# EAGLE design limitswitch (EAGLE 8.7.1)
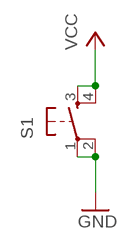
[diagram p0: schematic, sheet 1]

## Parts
S1  6MM_SWITCH6MM_SWITCH  [6MM_SWITCH]

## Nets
GND: S1.1(P) S1.2(P1)
VCC: S1.3(S) S1.4(S1)

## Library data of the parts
S1 = fab.lbr:6MM_SWITCH: OMRON SWITCH

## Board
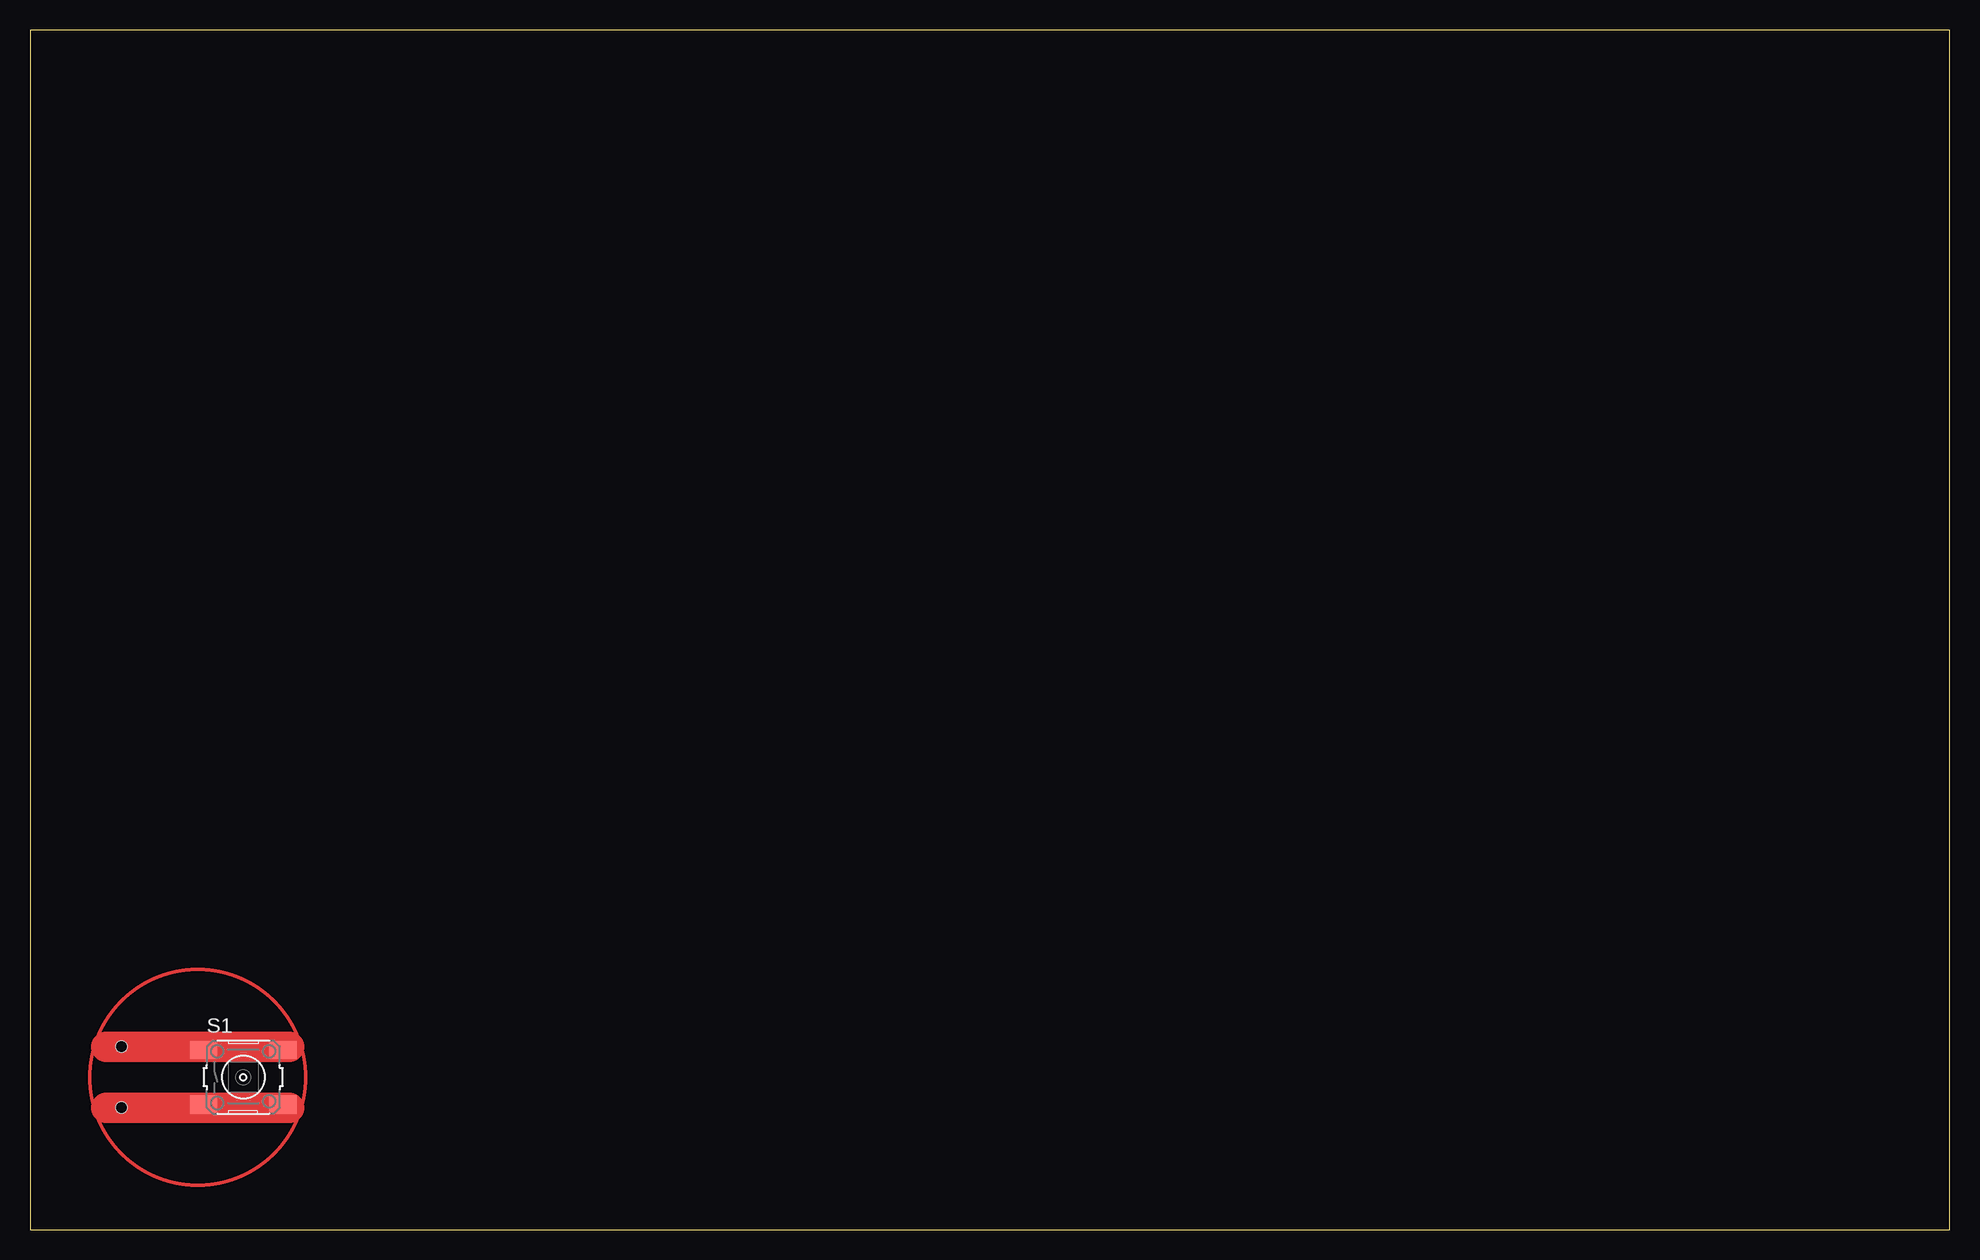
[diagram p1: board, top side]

Size 160 x 100 mm. Coordinates in mm from the lower left corner, seen from the top.
Outline: 0,0 160,0 160,100 0,100 0,0
Copper layers 1: Top 0.035mm
Design rules "basbasic": minimum track width 0.3mm, minimum drill 0.9mm, track to track 0.45mm, track to pad 0.45mm, pad to pad 0.45mm, via to via 0.45mm, smd to smd 6mil, copper to edge 40mil, drill to drill 6mil, minimum pad ring 10mil, minimum via ring 8mil, stop-mask expansion 4mil, vias tented up to drill 0mil, thermal gap 10mil
Holes 0.94 mm at 7.62,15.24 7.62,10.16

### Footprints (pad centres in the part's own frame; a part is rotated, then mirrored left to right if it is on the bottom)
6MM_SWITCH = smd 2.286 x 1.524: 1 -3.302,2.286; 2 3.302,2.286; 3 -3.302,-2.286; 4 3.302,-2.286

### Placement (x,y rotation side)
S1  17.78,12.7 0 top

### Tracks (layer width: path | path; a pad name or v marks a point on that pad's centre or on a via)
GND
  Top 0.305: S1.1 S1.2
N$1
  Top 2.54: 6.35,15.24 12.7,15.24 13.97,15.24 21.59,15.24
N$2
  Top 2.54: 6.35,10.16 12.7,10.16 13.97,10.16 21.59,10.16
VCC
  Top 0.305: S1.3 S1.4
(copper drawn outside any net)
  shapes: Top circle x1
